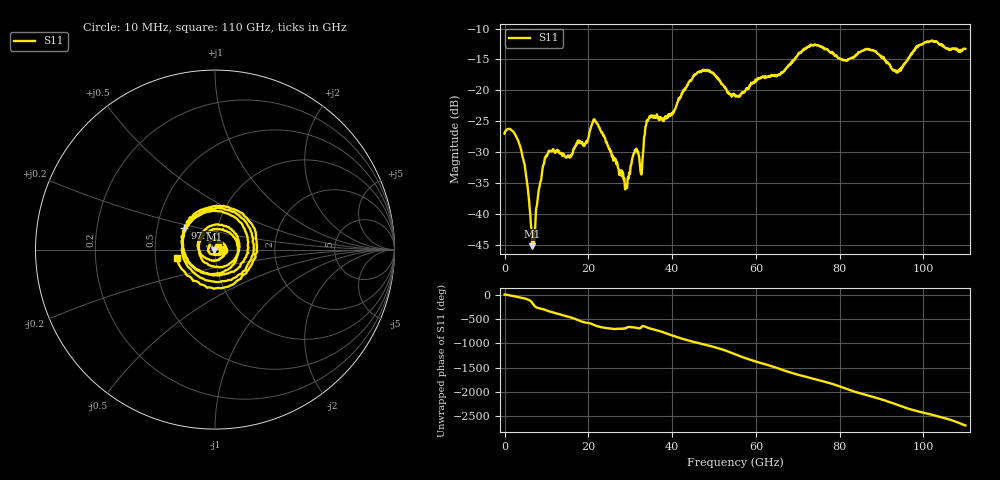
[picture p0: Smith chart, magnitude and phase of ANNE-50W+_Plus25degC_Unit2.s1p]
!Mini-Circuits Laboratory
!S-Parameters
!S1P File: Measurement
!Model: ANNE-50W+
!No.: Unit#2 (U2_25°C)
!Run / Lot / Date Code: QN2409253 /  / 2409
!Fixture: N/A
!Network Analyzer: PNA-X N5242B;  Serial number: 74314
!Pin Outs: PORT<1> = pin<1>
!TEST CONDITIONS: Z:50 OHM SYSTEM, INPUT POWER = 0dBm, TEMP:25°C
!F-F adapter to 1FT F-M cable on Port 2 head. 1mm 1 PORT SmartCal
!Date: 9/5/2024 at 12:58:23 PM
# Hz  S  dB  R  50
!Frequency  S11 dB  S11 Deg
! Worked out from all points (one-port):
!   2208 points, 10 MHz to 110 GHz, reference 50 ohm
!   lowest |S11| = -45.2 dB at 6.65 GHz (marker M1), VSWR 1.01, Z = 49.5 - j0.00324 ohm
!   |S11| at or under -10 dB: start of sweep to end of sweep
!   S11 on the Smith chart (normalised r, x): 10 MHz: 1.09, +0.00; 97.7 GHz: 0.69, +0.18; 110 GHz: 0.65, -0.06
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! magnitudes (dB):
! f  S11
! 10 MHz  -27.0
! 1.8 GHz  -26.5
! 3.7 GHz  -29.0
! 5.2 GHz  -34.1
! 6.65 GHz  -45.2
! 9.7 GHz  -30.9
! 13.8 GHz  -30.6
! 19.25 GHz  -28.6
! 21.6 GHz  -24.9
! 27.55 GHz  -33.0
! 29.15 GHz  -35.5
! 31.1 GHz  -29.7
! 32.65 GHz  -33.6
! 33.75 GHz  -25.7
! 34.45 GHz  -24.5
! 38.45 GHz  -24.1
! 41.3 GHz  -21.9
! 47.6 GHz  -16.8
! 55.05 GHz  -20.8
! 68.8 GHz  -15.2
! 73.55 GHz  -12.7
! 82.55 GHz  -14.8
! 87.55 GHz  -13.5
! 93.5 GHz  -16.9
! 96.3 GHz  -14.9
! 97.7 GHz  -13.6
! 102 GHz  -12.0
! 110 GHz  -13.3
